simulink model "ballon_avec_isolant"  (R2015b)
settings: Solver=ode23t  StartTime=0.0  StopTime=30000  RelTol=1e-3
libraries: fl_lib x7, nesl_utility x4

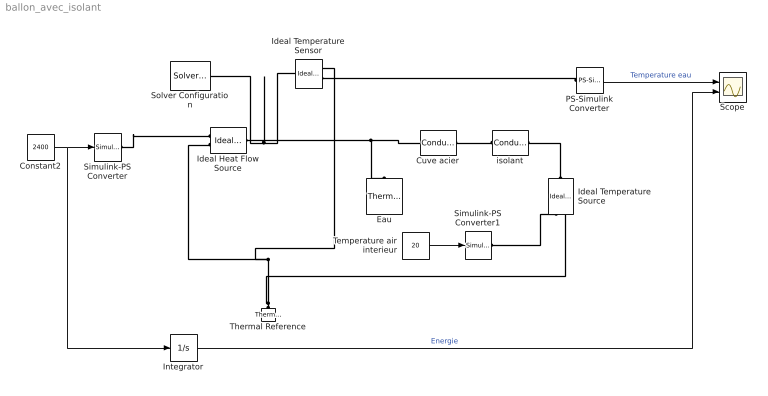
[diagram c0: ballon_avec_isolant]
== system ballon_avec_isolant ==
  Constant2 : Constant  Value=2400
  Cuve acier : fl_lib/Thermal/Thermal Elements/Conductive Heat Transfer  area=2.8 m^2  thickness=0.6 mm  th_cond=50 W/(m*K)  Q_specify=off  Q_priority=None  Q=0 J/s  T_specify=off  T_priority=None  T=0 K
  Eau : fl_lib/Thermal/Thermal Elements/Thermal Mass  mass=300 kg  sp_heat=4185 J/kg/K  Q_specify=off  Q_priority=None  Q=0 J/s  T_specify=on  T_priority=High  T=15 C
  Ideal Heat Flow Source : fl_lib/Thermal/Thermal Sources/Ideal Heat Flow Source
  Ideal Temperature Sensor : fl_lib/Thermal/Thermal Sensors/Ideal Temperature Sensor
  Ideal Temperature Source : fl_lib/Thermal/Thermal Sources/Ideal Temperature Source
  Integrator : Integrator
  PS-Simulink Converter : nesl_utility/PS-Simulink Converter  PhysicalDomain=network_engine_domain  SubClassName=ps_output  LeftPortType=input  RightPortType=output  PseudoPeriodic=off  Frequencies=[]  Unit=C  AffineConversion=on
  Scope : Scope  NumInputPorts=2
  Simulink-PS Converter : nesl_utility/Simulink-PS Converter  PhysicalDomain=network_engine_domain  SubClassName=ps_input  LeftPortType=input  RightPortType=output  PseudoPeriodic=off  Frequencies=[]  NoiseDistribution=none  NoiseParameters=[]  Unit=W  AffineConversion=on  InputFiltering=off  SimscapeFilterOrder=1  InputFilterTimeConstant=.001  UdotUserProvided=0
  Simulink-PS Converter1 : nesl_utility/Simulink-PS Converter  PhysicalDomain=network_engine_domain  SubClassName=ps_input  LeftPortType=input  RightPortType=output  PseudoPeriodic=off  Frequencies=[]  NoiseDistribution=none  NoiseParameters=[]  Unit=C  AffineConversion=on  InputFiltering=off  SimscapeFilterOrder=1  InputFilterTimeConstant=.001  UdotUserProvided=1
  Solver Configuration : nesl_utility/Solver Configuration  PhysicalDomain=network_engine_domain  SubClassName=solver  LeftPortType=input  RightPortType=generic  Accelerate=off  Tones=[]  Harmonics=[]  SimulateNoise=off  Profile=off  UseLocalSampling=off  EnableSwitchedLinearOptims=on  FrequencyDomain=off  UseCCode=off  RelTol=0.001  AbsTol=1e-06  MinStep=1e-09  ToWorkspace=off  RevertToSquareIcSolve=off  NumHomotopyIterations=100  PhasorMode=off  PhasorModeNumHarmonics=1  DoDC=off  ResidualTolerance=1e-09  UseLocalSolver=off  LocalSolverChoice=NE_BACKWARD_EULER_ADVANCER  LocalSolverSampleTime=0.001  DoFixedCost=off  MaxNonlinIter=3  MaxModeIter=2  LinearAlgebra=Sparse  DelaysMemoryBudget=1024  AutomaticFiltering=on  FilteringTimeConstant=0.001
  Temperature air interieur : Constant  Value=20
  Thermal Reference : fl_lib/Thermal/Thermal Elements/Thermal Reference
  isolant : fl_lib/Thermal/Thermal Elements/Conductive Heat Transfer  area=0 m^2  thickness=0 mm  th_cond=0 W/(m*K)  Q_specify=off  Q_priority=None  Q=0 J/s  T_specify=off  T_priority=None  T=0 K
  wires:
  PS-Simulink Converter/1 -> Scope/1  "Temperature eau"
  Integrator/1 -> Scope/2  "Energie"
  Temperature air interieur/1 -> Simulink-PS Converter1/1
  Constant2/1 -> Simulink-PS Converter/1, Integrator/1
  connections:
  Ideal Heat Flow Source/LConn1 -- Cuve acier/LConn1 -- Eau/LConn1 -- Solver Configuration/RConn1 -- Ideal Temperature Sensor/LConn1
  Thermal Reference/LConn1 -- Ideal Temperature Source/RConn2 -- Ideal Temperature Sensor/RConn1 -- Ideal Heat Flow Source/RConn2
  Simulink-PS Converter/RConn1 -- Ideal Heat Flow Source/RConn1
  PS-Simulink Converter/LConn1 -- Ideal Temperature Sensor/RConn2
  Ideal Temperature Source/LConn1 -- isolant/RConn1
  Simulink-PS Converter1/RConn1 -- Ideal Temperature Source/RConn1
  isolant/LConn1 -- Cuve acier/RConn1
